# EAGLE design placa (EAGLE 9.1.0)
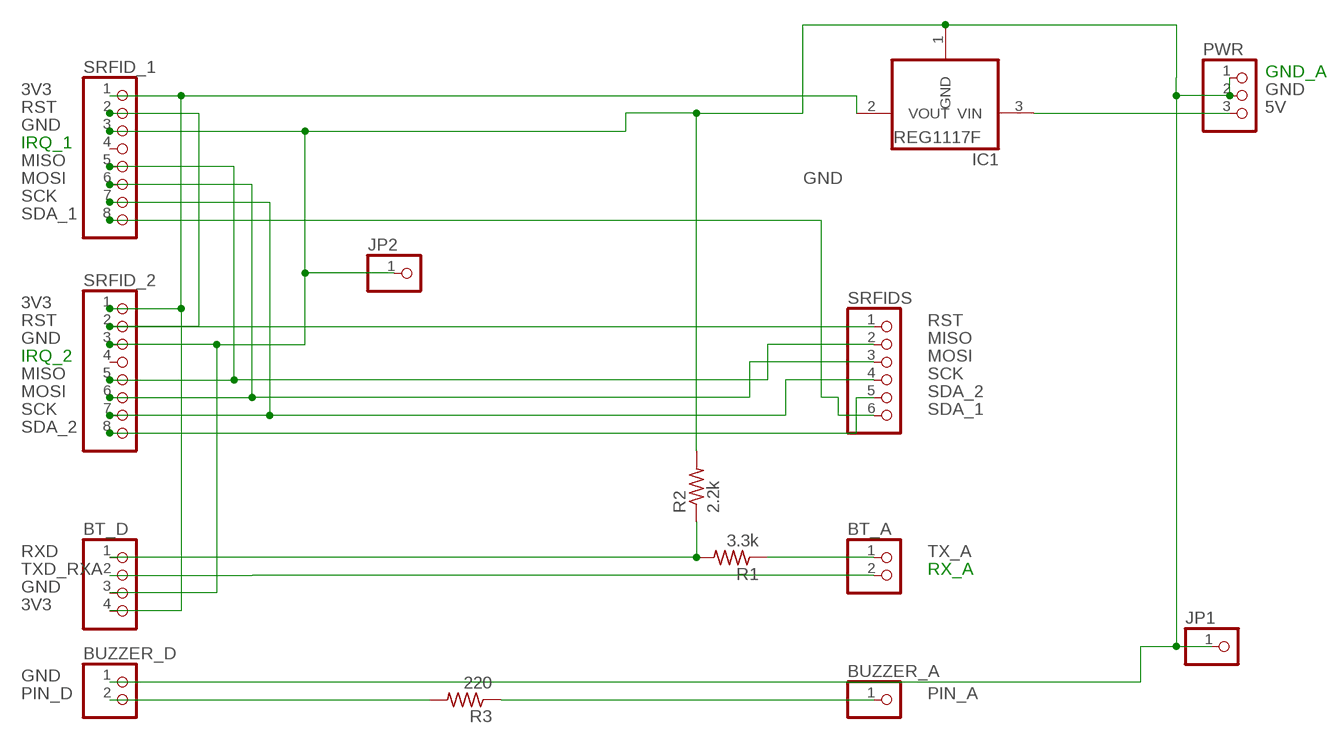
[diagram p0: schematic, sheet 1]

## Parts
BT_A  PINHD-1X2  [1X02]
BT_D  PINHD-1X4  [1X04]
BUZZER_A  PINHD-1X1  [1X01]
BUZZER_D  PINHD-1X2  [1X02]
IC1  REG1117F  [DD-3]
JP1  PINHD-1X1  [1X01]
JP2  PINHD-1X1  [1X01]
PWR  PINHD-1X3  [1X03]
R1  3.3k  R-US_0207/10  [0207/10]
R2  2.2k  R-US_0207/10  [0207/10]
R3  220  R-US_0207/10  [0207/10]
SRFID_1  PINHD-1X8  [1X08]
SRFID_2  PINHD-1X8  [1X08]
SRFIDS  PINHD-1X6  [1X06]

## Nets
3V3: BT_D.4 IC1.2(VOUT) SRFID_1.1 SRFID_2.1
5V: IC1.3(VIN) PWR.3
GND: BT_D.3 BUZZER_D.1 IC1.1(GND) JP1.1 JP2.1 PWR.1 PWR.2 R2.2 SRFID_1.3 SRFID_2.3
MISO: SRFID_1.5 SRFID_2.5 SRFIDS.2
MOSI: SRFID_1.6 SRFID_2.6 SRFIDS.3
PIN_A: BUZZER_A.1 R3.1
PIN_D: BUZZER_D.2 R3.2
RST: SRFID_1.2 SRFID_2.2 SRFIDS.1
RXD: BT_D.1 R1.2 R2.1
SCK: SRFID_1.7 SRFID_2.7 SRFIDS.4
SDA_1: SRFID_1.8 SRFIDS.6
SDA_2: SRFID_2.8 SRFIDS.5
TX_A: BT_A.1 R1.1
TXD_RXA: BT_A.2 BT_D.2
Unconnected: SRFID_1.4 SRFID_2.4

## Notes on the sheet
- GND_A
- IRQ_1
- IRQ_2
- RX_A

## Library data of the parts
BT_A BUZZER_D = pinhead:PINHD-1X2: PIN HEADER
BT_D = pinhead:PINHD-1X4: PIN HEADER
BUZZER_A JP1 JP2 = pinhead:PINHD-1X1: PIN HEADER
IC1 = burr-brown:REG1117: 800mA and 1A Low Dropout (LDO) Positive Regulator 1.8V, 2.5V, 2.85V, 3.3V, 5V, and Adj; MF: TEXAS INSTRUMENTS; MPN: REG1117FAKTTT; OC_FARNELL: 1296120; OC_NEWARK: 87H2562
PWR = pinhead:PINHD-1X3: PIN HEADER
R1-R3 = rcl:R-US_: RESISTOR, American symbol; SPICEPREFIX: R
SRFID_1 SRFID_2 = pinhead:PINHD-1X8: PIN HEADER
SRFIDS = pinhead:PINHD-1X6: PIN HEADER

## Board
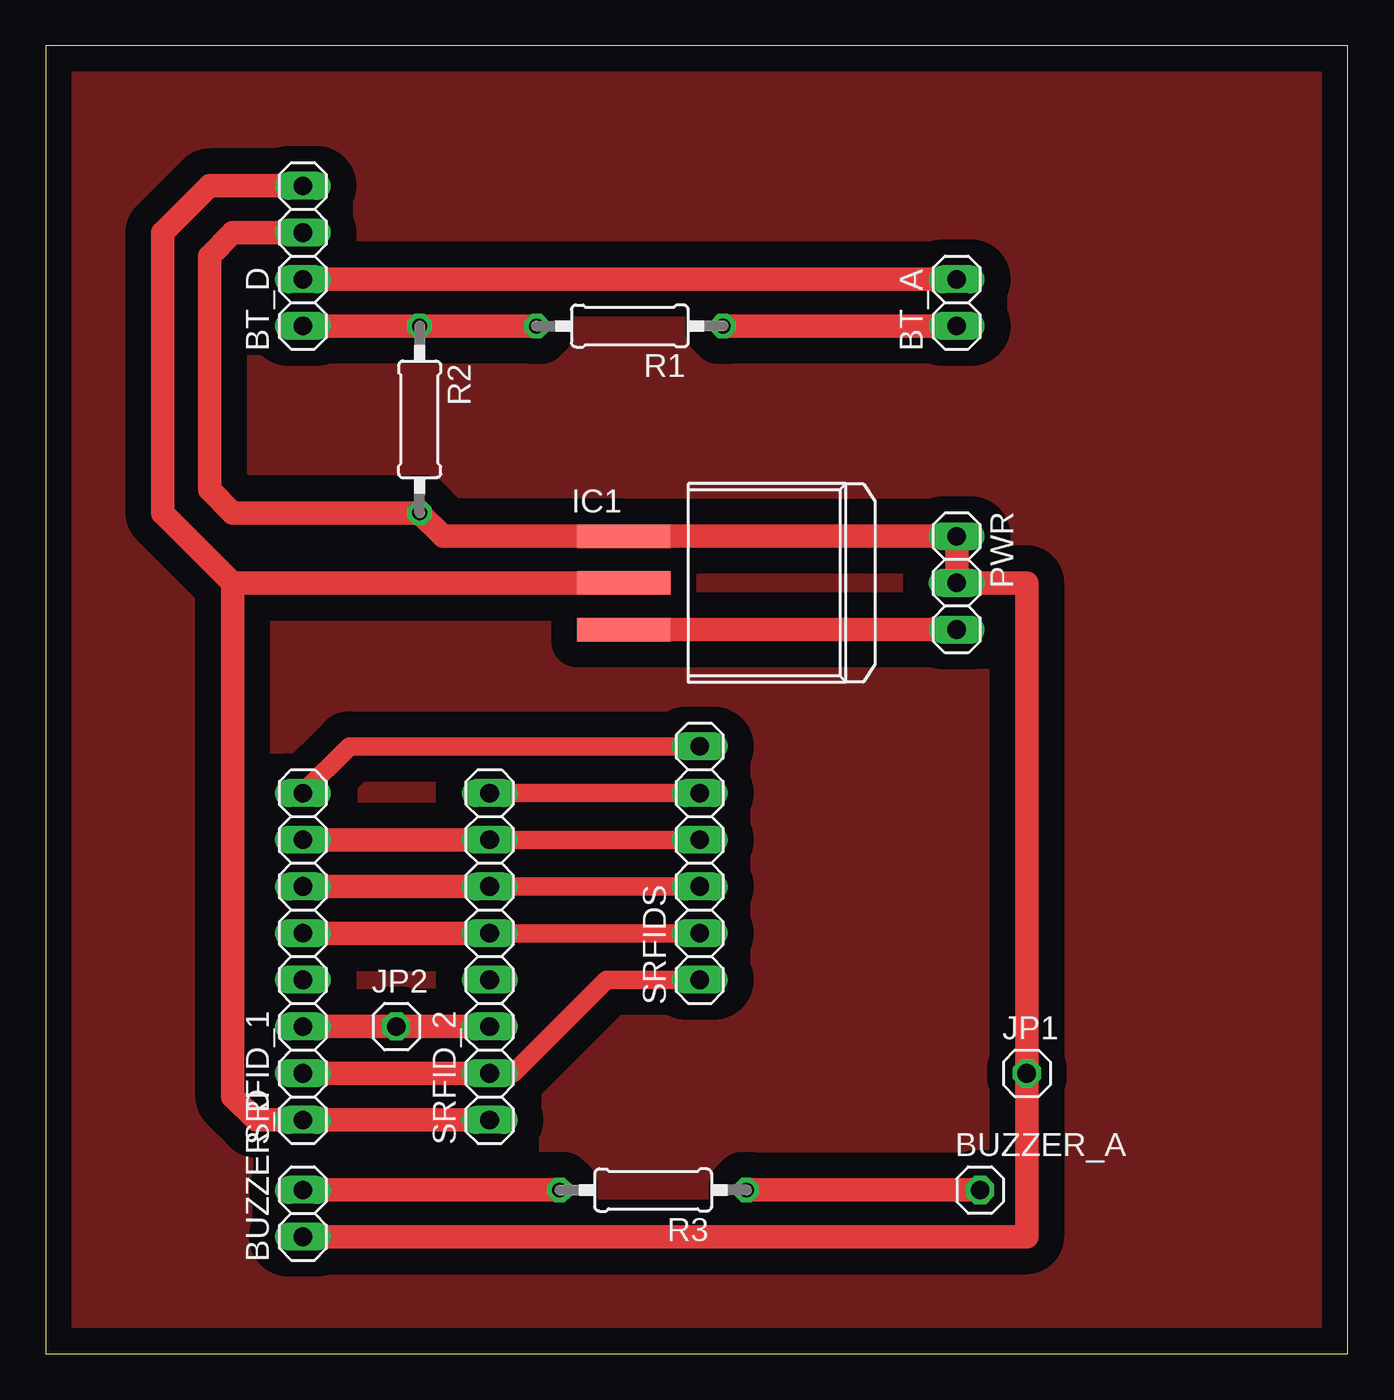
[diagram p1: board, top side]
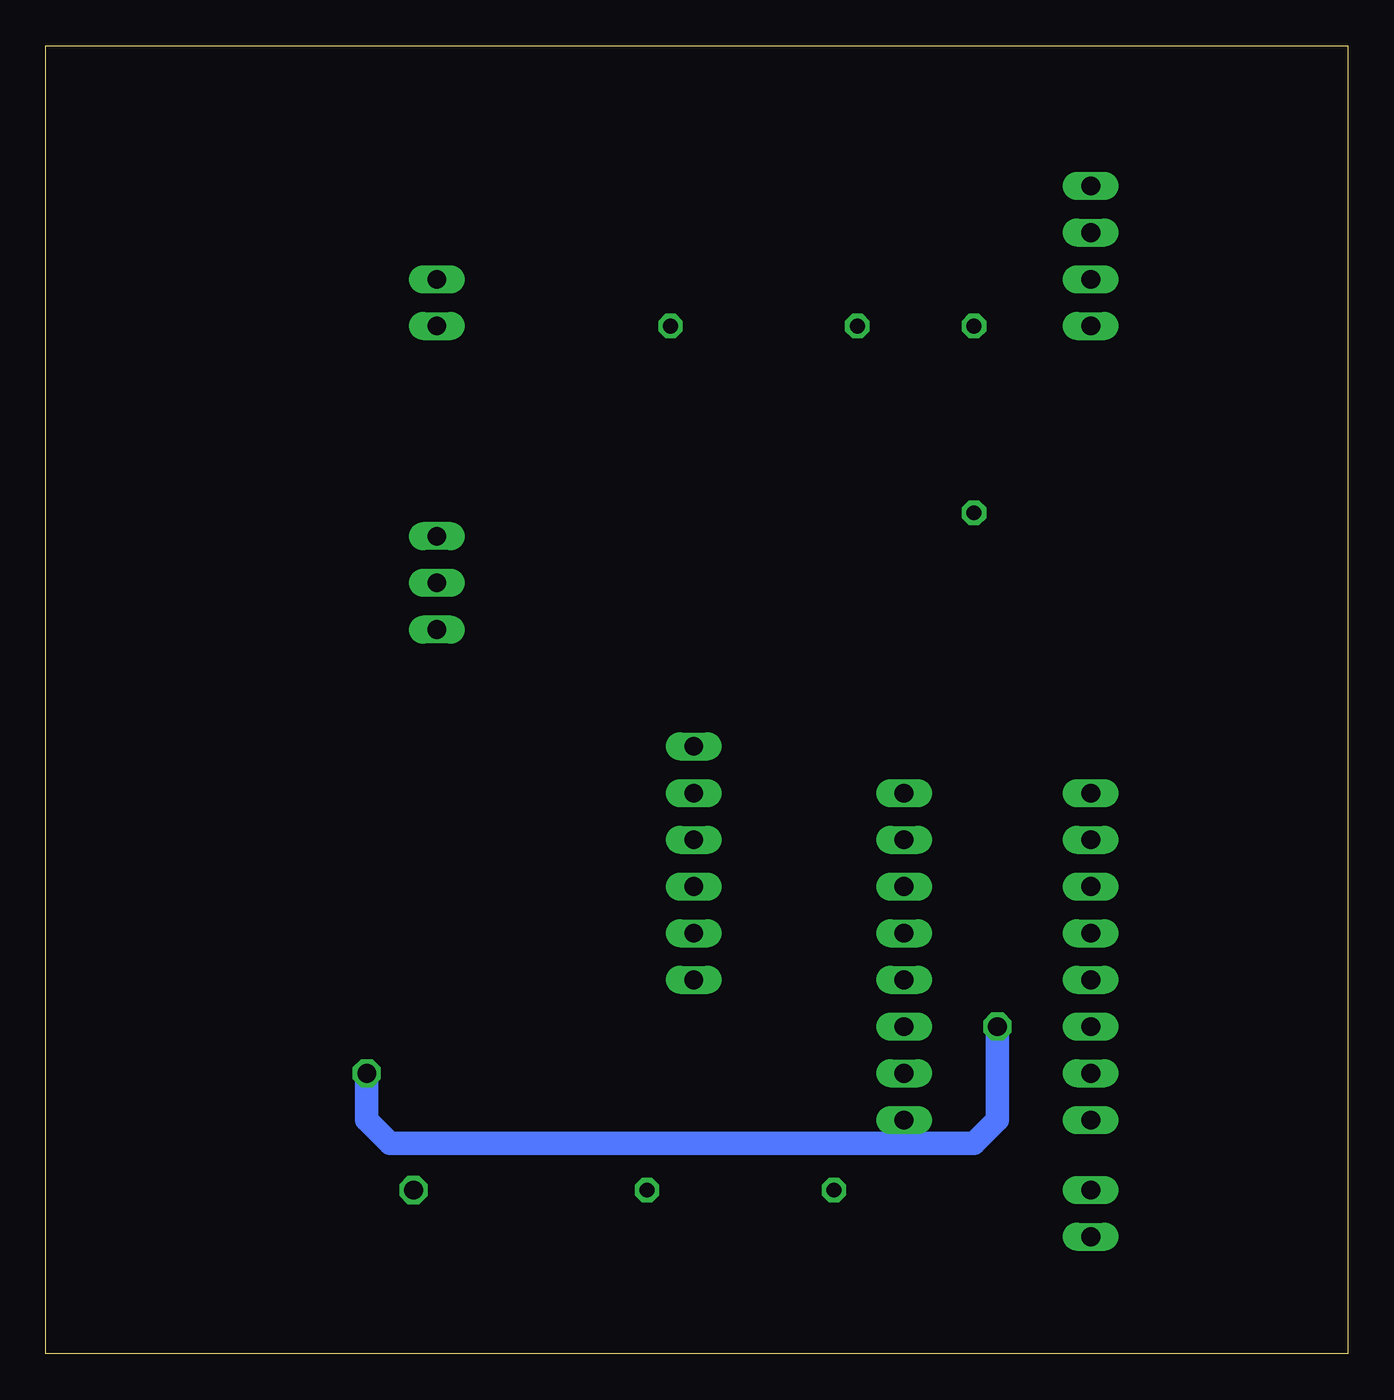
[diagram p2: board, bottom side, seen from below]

Size 70.79 x 71.11 mm. Coordinates in mm from the lower left corner, seen from the top.
Outline: 0,0 70.79,0 70.79,71.11 0,71.11 0,0
Copper layers (1*16): Top 0.035mm / dielectric 2mm / Bottom 0.035mm
Design rules "default *": minimum track width 6mil, minimum drill 0.35mm, track to track 10mil, track to pad 10mil, pad to pad 10mil, via to via 10mil, smd to smd 6mil, copper to edge 40mil, drill to drill 6mil, minimum pad ring 10mil, minimum via ring 8mil, stop-mask expansion 4mil, vias tented up to drill 0mil, thermal gap 10mil

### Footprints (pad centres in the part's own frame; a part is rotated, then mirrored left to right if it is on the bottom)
1X02 = drill 1.016 long: 1 -1.27,0; 2 1.27,0
1X04 = drill 1.016 long: 1 -3.81,0; 2 -1.27,0; 3 1.27,0; 4 3.81,0
1X01 = drill 1.016 octagon: 1 0,0
DD-3 = smd 1.27 x 5.08: 1 -2.54,-7.938; 2 0,-7.938; 3 2.54,-7.938
1X03 = drill 1.016 long: 1 -2.54,0; 2 0,0; 3 2.54,0
0207/10 = drill 0.813 octagon: 1 -5.08,0; 2 5.08,0
1X08 = drill 1.016 long: 1 -8.89,0; 2 -6.35,0; 3 -3.81,0; 4 -1.27,0; 5 1.27,0; 6 3.81,0; 7 6.35,0; 8 8.89,0
1X06 = drill 1.016 long: 1 -6.35,0; 2 -3.81,0; 3 -1.27,0; 4 1.27,0; 5 3.81,0; 6 6.35,0

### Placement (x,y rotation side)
BT_A  49.53,57.15 90 top
BT_D  13.97,59.69 90 top
BUZZER_A  50.8,8.89 0 top
BUZZER_D  13.97,7.62 90 top
IC1  39.37,41.91 270 top
JP1  53.34,15.24 0 top
JP2  19.05,17.78 0 top
PWR  49.53,41.91 270 top
R1  31.75,55.88 180 top
R2  20.32,50.8 270 top
R3  33.02,8.89 180 top
SRFID_1  13.97,21.59 90 top
SRFID_2  24.13,21.59 90 top
SRFIDS  35.56,26.67 90 top

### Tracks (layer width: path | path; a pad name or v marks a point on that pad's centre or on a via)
3V3
  Top 1.27: BT_D.4 8.89,63.5 6.35,60.96 6.35,45.72 10.16,41.91 | 10.16,41.91 IC1.2 | SRFID_2.1 SRFID_1.1 11.43,12.7 10.16,13.97 10.16,41.91 | 10.16,41.91
5V
  Top 1.27: IC1.3 PWR.3
GND
  Top 1.27: BT_D.3 10.16,60.96 8.89,59.69 8.89,46.99 10.16,45.72 R2.2 21.59,44.45 IC1.1 PWR.1 PWR.2 53.34,41.91 JP1.1 53.34,6.35 BUZZER_D.1 | SRFID_1.3 JP2.1 SRFID_2.3
  Bottom 1.27: JP2.1 19.05,12.7 20.32,11.43 52.07,11.43 53.34,12.7 JP1.1
KK
  pour Top (isolate 1.397): 1.27,69.85 1.27,1.27 69.85,1.27 69.85,69.85
MISO
  Top 1.016: SRFID_2.5 SRFIDS.2
  Top 1.27: SRFID_1.5 SRFID_2.5
MOSI
  Top 1.016: SRFID_2.6 SRFIDS.3
  Top 1.27: SRFID_1.6 SRFID_2.6
PIN_A
  Top 1.27: R3.1 BUZZER_A.1
PIN_D
  Top 1.27: R3.2 BUZZER_D.2
RST
  Top 1.016: SRFIDS.1 30.48,20.32 25.4,15.24 SRFID_2.2
  Top 1.27: SRFID_1.2 SRFID_2.2
RXD
  Top 1.27: R1.2 R2.1 BT_D.1
SCK
  Top 1.016: SRFID_2.7 SRFIDS.4
  Top 1.27: SRFID_1.7 SRFID_2.7
SDA_1
  Top 1.016: SRFID_1.8 16.51,33.02 SRFIDS.6
SDA_2
  Top 1.016: SRFID_2.8 SRFIDS.5
TX_A
  Top 1.27: BT_A.1 R1.1
TXD_RXA
  Top 1.27: BT_A.2 BT_D.2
